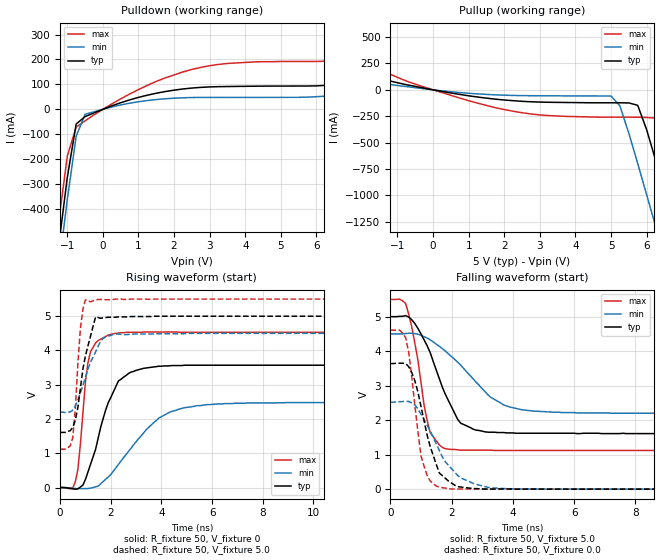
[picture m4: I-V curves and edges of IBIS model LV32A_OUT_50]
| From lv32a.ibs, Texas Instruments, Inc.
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|   Model LV32A_OUT_50
[Model]   LV32A_OUT_50
Model_type  Output
Polarity   Non-Inverting
Vmeas = 2.50v
Cref = 15pf
| variable   typ   min   max
C_comp   4.62pf   3.47pf   5.77pf
[Temperature Range]   25   85   -40
[Voltage Range]   5.0   4.5   5.5
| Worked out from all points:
|   slope of the pulldown table from 0 to 0.75 V, typ, clamps not added: 19.9 ohm
|   slope of the pullup table from 0 to 0.75 V, typ, clamps not added: 17.2 ohm
|   rising waveform, R_fixture 50, V_fixture 0: 20-80 % time 925ps typ, 1.72ns min, 345ps max; typ from 0 V to 3.57 V
|   falling waveform, R_fixture 50, V_fixture 5.0: 20-80 % time 946ps typ, 1.54ns min, 485ps max; typ from 5 V to 1.61 V
|   rising waveform, R_fixture 50, V_fixture 5.0: 20-80 % time 479ps typ, 700ps min, 235ps max; typ from 1.61 V to 5 V
|   falling waveform, R_fixture 50, V_fixture 0.0: 20-80 % time 624ps typ, 986ps min, 377ps max; typ from 3.64 V to 0 V
[Pulldown]
|   Voltage   I(typ)   I(min)   I(max)
-5V       -5.14A     -5.22A     -5.05A
-1.5V     -853mA     -945mA     -756mA
-1.25V    -557mA     -649mA     -461mA
-1V       -274mA     -363mA     -188mA
-750mV    -58.9mA    -108mA     -71.3mA
-500mV    -29.2mA    -20mA      -46.2mA
0V        -3.33nA    -3.4nA     -3.57nA
1.25V     56.7mA     35.2mA     96mA
2.5V      85.3mA     47.3mA     160mA
3.5V      91.4mA     47.8mA     184mA
6.75V     103mA      58.5mA     199mA
10V       179mA      107mA      329mA
[Pullup]
|   Voltage   I(typ)   I(min)   I(max)
-5V       310mA      167mA      586mA
-3.5V     252mA      143mA      464mA
-750mV    48.6mA     30.8mA     83.5mA
1.5V      -78.8mA    -43.4mA    -148mA
5V        -123mA     -58.9mA    -259mA
5.25V     -123mA     -153mA     -259mA
5.75V     -147mA     -699mA     -260mA
6.25V     -664mA     -1.29A     -268mA
6.5V      -960mA     -1.6A      -403mA
6.75V     -1.26A     -1.9A      -685mA
7.25V     -1.87A     -2.51A     -1.28A
10V       -5.25A     -5.89A     -4.66A
[Ramp]
| variable   typ   min   max
dV/dt_r   2.15E+00/8.45E-10   1.50E+00/1.75E-09   2.73E+00/3.33E-10
dV/dt_f   2.05E+00/9.33E-10   1.39E+00/1.55E-09   2.64E+00/5.19E-10
R_load = 50
[Rising Waveform]
R_fixture = 50
V_fixture = 0
|   Time   V(typ)   V(min)   V(max)
0s        0V         0V         0V
600ps     -45.8mV    -25.9mV    171mV
700ps     -36.3mV    -28.9mV    534mV
1ns       241mV      -28.5mV    3.1V
1.2ns     679mV      -17.3mV    3.97V
2.1ns     2.79V      477mV      4.49V
2.7ns     3.33V      1.06V      4.53V
3.9ns     3.54V      2.03V      4.54V
5.4ns     3.57V      2.39V      4.53V
25ns      3.57V      2.48V      4.53V
[Falling Waveform]
R_fixture = 50
V_fixture = 5.0
V_fixture_min = 4.5
V_fixture_max = 5.5
|   Time   V(typ)   V(min)   V(max)
0s        5V         4.5V       5.5V
500ps     5.03V      4.51V      5.38V
700ps     4.91V      4.52V      4.7V
1.3ns     3.96V      4.33V      1.64V
1.8ns     2.74V      4V         1.17V
2.2ns     2.02V      3.68V      1.14V
2.7ns     1.74V      3.2V       1.13V
3.7ns     1.64V      2.44V      1.12V
4.7ns     1.62V      2.26V      1.12V
25ns      1.61V      2.2V       1.12V
[Rising Waveform]
R_fixture = 50
V_fixture = 5.0
V_fixture_min = 4.5
V_fixture_max = 5.5
|   Time   V(typ)   V(min)   V(max)
0s        1.61V      2.2V       1.12V
400ps     1.66V      2.21V      1.22V
500ps     1.76V      2.26V      1.46V
600ps     1.97V      2.38V      2.32V
800ps     2.9V       2.76V      4.65V
1ns       3.85V      3.22V      5.48V
1.4ns     4.98V      3.96V      5.47V
1.7ns     4.95V      4.36V      5.49V
2.2ns     4.97V      4.48V      5.5V
25ns      5V         4.5V       5.5V
[Falling Waveform]
R_fixture = 50
V_fixture = 0.0
|   Time   V(typ)   V(min)   V(max)
0s        3.64V      2.52V      4.61V
500ps     3.64V      2.55V      4.39V
600ps     3.55V      2.54V      3.96V
800ps     3.14V      2.44V      2.42V
1ns       2.4V       2.17V      969mV
1.3ns     1.24V      1.69V      236mV
1.6ns     467mV      1.12V      53.8mV
2.3ns     61.2mV     327mV      5.08mV
3.7ns     6.18mV     17.1mV     971uV
25ns      9.21uV     2.64uV     9.49uV
